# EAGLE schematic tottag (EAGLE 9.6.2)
AUTHOR: Andreas Biri & Pat Pannuto; REV: G; TITLE: TotTag

## Sheet 1 of 4: nRF8240
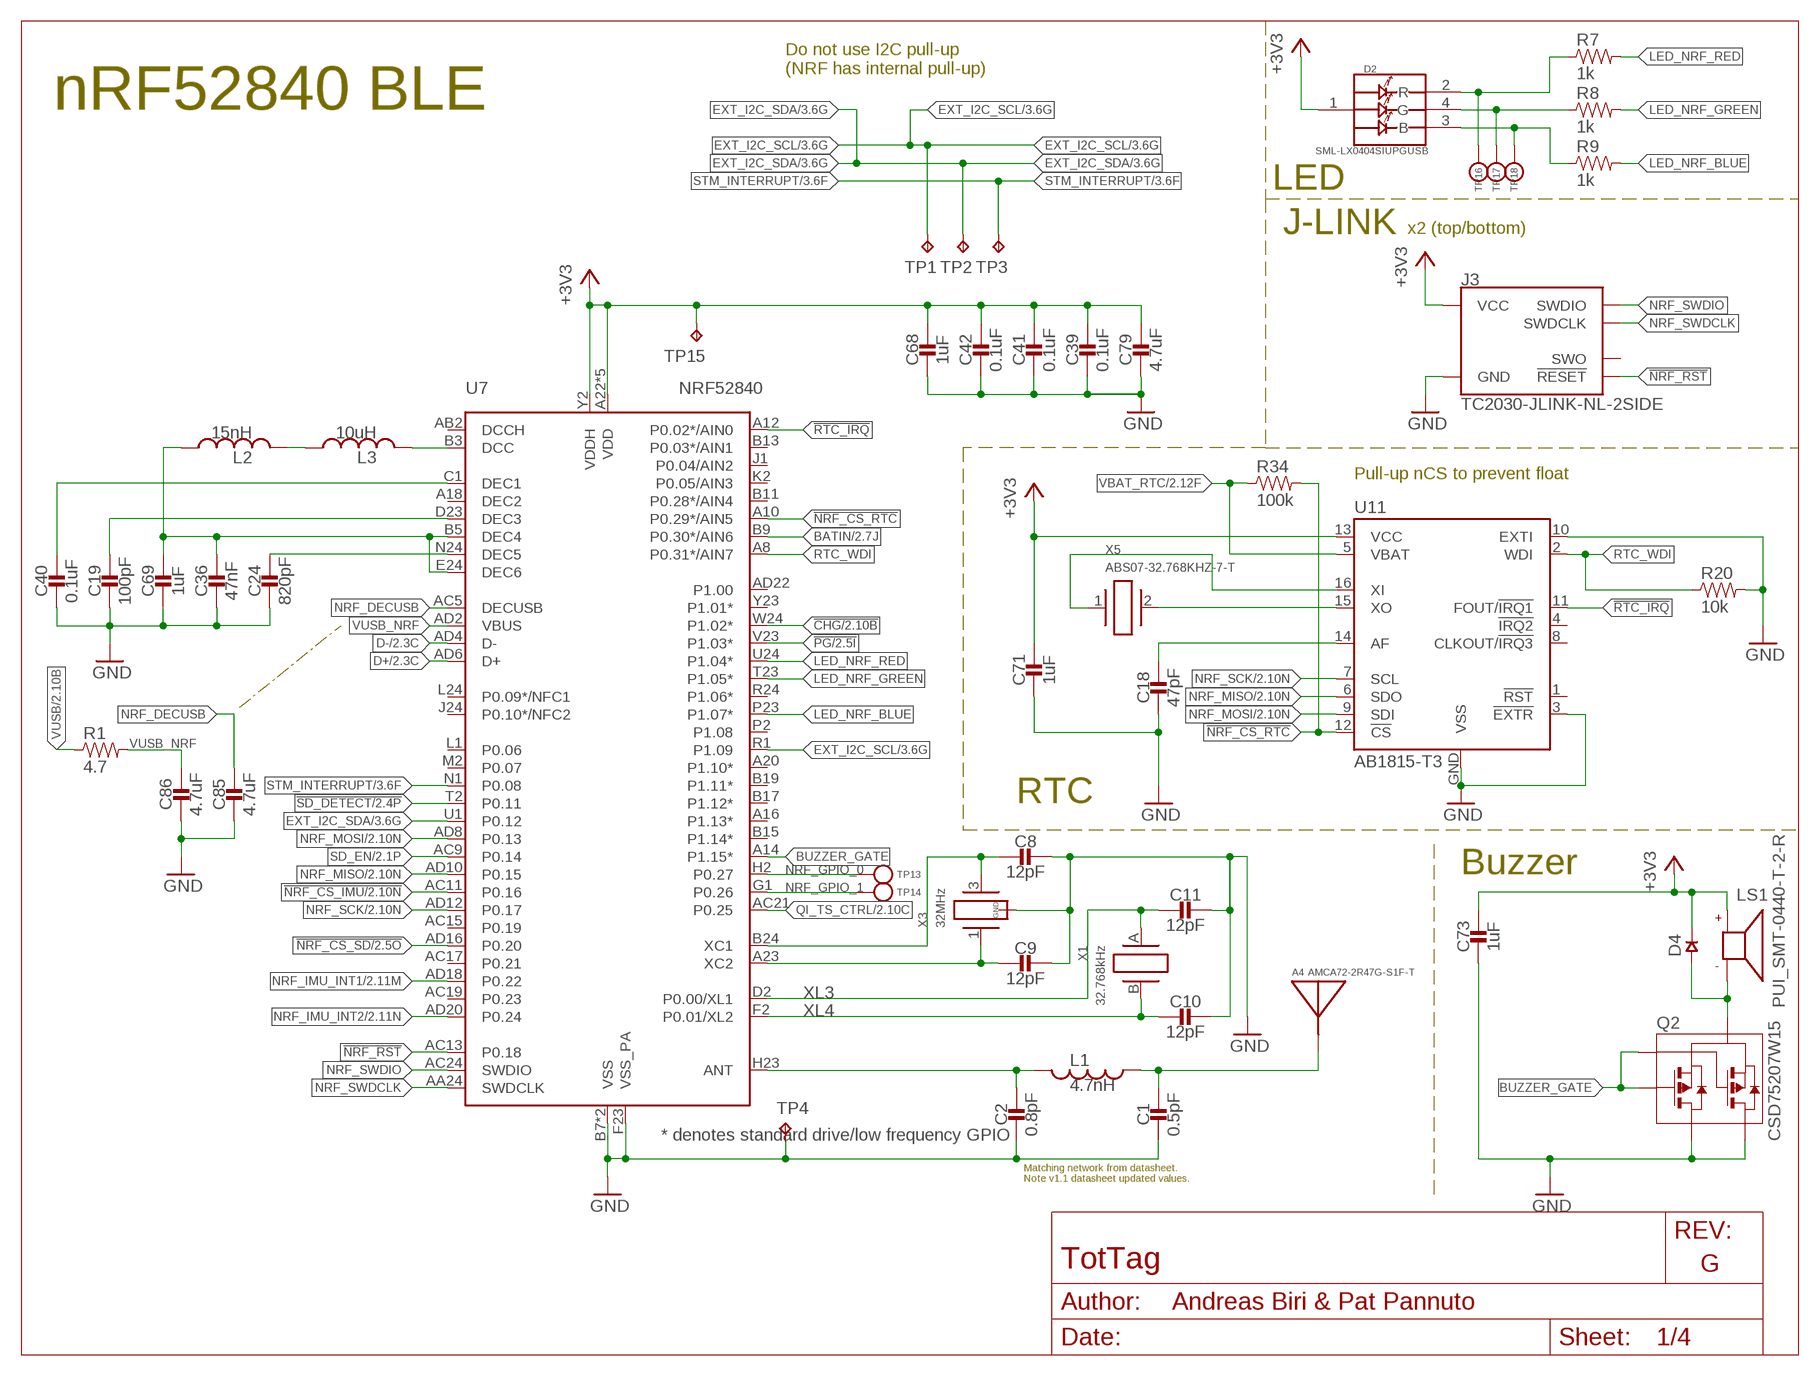
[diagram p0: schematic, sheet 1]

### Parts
A4  AMCA72-2R47G-S1F-T  [AMCA72-2R470G-S1F-T]
C1  0.5pF  CAPACITOR0402_CAP  [0402_CAP]
C2  0.8pF  CAPACITOR0402_CAP  [0402_CAP]
C8  12pF  CAPACITOR0402_CAP  [0402_CAP]
C9  12pF  CAPACITOR0402_CAP  [0402_CAP]
C10  12pF  CAPACITOR0402_CAP  [0402_CAP]
C11  12pF  CAPACITOR0402_CAP  [0402_CAP]
C18  47pF  CAPACITOR0402_CAP  [0402_CAP]
C19  100pF  CAPACITOR0402_CAP  [0402_CAP]
C24  820pF  CAPACITOR0402_CAP  [0402_CAP]
C36  47nF  CAPACITOR0402_CAP  [0402_CAP]
C39  0.1uF  CAPACITOR0402_CAP  [0402_CAP]
C40  0.1uF  CAPACITOR0402_CAP  [0402_CAP]
C41  0.1uF  CAPACITOR0402_CAP  [0402_CAP]
C42  0.1uF  CAPACITOR0402_CAP  [0402_CAP]
C68  1uF  CAPACITOR0402_CAP  [0402_CAP]
C69  1uF  CAPACITOR0402_CAP  [0402_CAP]
C71  1uF  CAPACITOR0402_CAP  [0402_CAP]
C73  1uF  CAPACITOR0402_CAP  [0402_CAP]
C79  4.7uF  CAPACITOR0402_CAP  [0402_CAP]
C85  4.7uF  CAPACITOR0402_CAP  [0402_CAP]
C86  4.7uF  CAPACITOR0402_CAP  [0402_CAP]
D2  SML-LX0404SIUPGUSB  [1MM_SQ_4PAD]
D4  DIODE0402  [0402_DIODE]
J3  TC2030-JLINK-NL-2SIDE  [TC2030-IDC-NL-2SIDE]
L1  4.7nH  INDUCTOR0402  [0402_CAP]
L2  15nH  INDUCTOR0402  [0402_CAP]
L3  10uH  INDUCTOR0603  [0603_CAP]
LS1  PUI_SMT-0440-T-2-R  [SMT-0440-T-2-R]
Q2  CSD75207W15  [DSBGA]
R1  4.7  RESISTOR0402_RES  [0402_RES]
R7  1k  RESISTOR0402_RES  [0402_RES]
R8  1k  RESISTOR0402_RES  [0402_RES]
R9  1k  RESISTOR0402_RES  [0402_RES]
R20  10k  RESISTOR0402_RES  [0402_RES]
R34  100k  RESISTOR0402_RES  [0402_RES]
TP1  TPTP06SQ  [TP06SQ]
TP2  TPTP06SQ  [TP06SQ]
TP3  TPTP06SQ  [TP06SQ]
TP4  TPTP06SQ  [TP06SQ]
TP13  TEST-POINT  [PAD.03X.03]
TP14  TEST-POINT  [PAD.03X.03]
TP15  TPTP06SQ  [TP06SQ]
TP16  TEST-POINT  [PAD.03X.03]
TP17  TEST-POINT  [PAD.03X.03]
TP18  TEST-POINT  [PAD.03X.03]
U7  NRF52840  [AQFN73]
U11  AB1815-T3  [QFN-16-3MM]
X1  32.768kHz  ABS05-32.768KHZ-9-T  [ABS05]
X3  32MHz  7V-32.000MAHV-T  [TXC-7V]
X5  ABS07-32.768KHZ-7-T  [ABS07]

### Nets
!CHG: U7.W24(P1.02*) ; also sheet 2
!NRF_CS_IMU: U7.AC11(P0.16) ; also sheet 2
!NRF_CS_RTC: R34.2 U7.A10(P0.29*/AIN5) U11.12(!CS)
!NRF_CS_SD: U7.AD16(P0.20) ; also sheet 2
!NRF_RST: J3.3(!RESET) J3.B3(!RESET) U7.AC13(P0.18)
!PG: U7.V23(P1.03*) ; also sheet 2
!RTC_IRQ: U7.A12(P0.02*/AIN0) U11.11(FOUT/!IRQ1)
!SD_DETECT: U7.T2(P0.11) ; also sheet 2
+3V3: C39.1 C41.1 C42.1 C68.1 C71.1 C73.1 C79.1 D2.1(VDD) D4.CATHODE J3.1(VCC) J3.B1(VCC) LS1.+(P) TP15.TP U7.A22(VDD) U7.AD14(VDD) U7.AD23(VDD) U7.B1(VDD) U7.W1(VDD) U7.Y2(VDDH) U11.13(VCC) ; also sheet 2,3,4
BATIN: U7.B9(P0.30*/AIN6) ; also sheet 2
BLE_ANT: A4.S1(ANTENNA) C1.1 L1.1
BUZZER_GATE: Q2.A1(G1) Q2.C1(G2) U7.A14(P1.15*)
D+: U7.AD6(D+) ; also sheet 2
D-: U7.AD4(D-) ; also sheet 2
EXT_I2C_SCL: TP1.TP U7.R1(P1.09) ; also sheet 3,4
EXT_I2C_SDA: TP2.TP U7.U1(P0.12) ; also sheet 3,4
GND: C1.2 C2.2 C8.1 C9.1 C10.1 C11.1 C18.2 C19.2 C24.2 C36.2 C39.2 C40.2 C41.2 C42.2 C68.2 C69.2 C71.2 C73.2 C79.2 C85.2 C86.2 J3.5(GND) J3.B5(GND) Q2.A2(D1) Q2.A3(D1) Q2.B2(D2) Q2.B3(D1) Q2.C2(D2) Q2.C3(D2) R20.2 TP4.TP U7.B7(VSS) U7.F23(VSS_PA) U7.GND(VSS) U11.3(!EXTR) U11.10(EXTI) U11.GND(VSS) X3.2(GND) X3.4(GND) ; also sheet 2,3
LED_NRF_BLUE: R9.2 U7.P23(P1.07*)
LED_NRF_GREEN: R8.2 U7.T23(P1.05*)
LED_NRF_RED: R7.2 U7.U24(P1.04*)
N$2: D4.ANODE LS1.-(N) Q2.B1(S)
N$15: C2.1 L1.2 U7.H23(ANT)
N$18: C8.2 U7.B24(XC1) X3.3
N$19: C9.2 U7.A23(XC2) X3.1
N$35: C18.1 U11.14(AF)
N$37: L2.2 L3.1
N$41: U11.16(XI) X5.1
N$42: U11.15(XO) X5.2
N$59: D2.2(R) R7.1 TP16.P$1(TESTPOINT)
N$60: D2.4(G) R8.1 TP17.P$1(TESTPOINT)
N$61: D2.3(B) R9.1 TP18.P$1(TESTPOINT)
NRF_DCC: L3.2 U7.B3(DCC)
NRF_DECAP1: C40.1 U7.C1(DEC1)
NRF_DECAP3: C19.1 U7.D23(DEC3)
NRF_DECAP5: C24.1 U7.N24(DEC5)
NRF_DECAP46: C36.1 C69.1 L2.1 U7.B5(DEC4) U7.E24(DEC6)
NRF_DECUSB: C85.1 U7.AC5(DECUSB)
NRF_GPIO_0: TP13.P$1(TESTPOINT) U7.H2(P0.27)
NRF_GPIO_1: TP14.P$1(TESTPOINT) U7.G1(P0.26)
NRF_IMU_INT1: U7.AD18(P0.22) ; also sheet 2
NRF_IMU_INT2: U7.AD20(P0.24) ; also sheet 2
NRF_MISO: U7.AD10(P0.15) U11.6(SDO) ; also sheet 2
NRF_MOSI: U7.AD8(P0.13) U11.9(SDI) ; also sheet 2
NRF_SCK: U7.AD12(P0.17) U11.7(SCL) ; also sheet 2
NRF_SWDCLK: J3.4(SWDCLK) J3.B4(SWDCLK) U7.AA24(SWDCLK)
NRF_SWDIO: J3.2(SWDIO) J3.B2(SWDIO) U7.AC24(SWDIO)
QI_TS_CTRL: U7.AC21(P0.25) ; also sheet 2
RTC_WDI: R20.1 U7.A8(P0.31*/AIN7) U11.2(WDI)
SD_EN: U7.AC9(P0.14) ; also sheet 2
STM_INTERRUPT: TP3.TP U7.N1(P0.08) ; also sheet 3,4
VBAT_RTC: R34.1 U11.5(VBAT) ; also sheet 2
VUSB: R1.1 ; also sheet 2
VUSB_NRF: C86.1 R1.2 U7.AD2(VBUS)
XL3: C11.2 U7.D2(P0.00/XL1) X1.A
XL4: C10.2 U7.F2(P0.01/XL2) X1.B
Unconnected: J3.6(SWO) J3.B6(SWO) U7.A16(P1.13*) U7.A18(DEC2) U7.A20(P1.10*) U7.AB2(DCCH) U7.AC15(P0.19) U7.AC17(P0.21) U7.AC19(P0.23) U7.AD22(P1.00) U7.B11(P0.28*/AIN4) U7.B13(P0.03*/AIN1) U7.B15(P1.14*) U7.B17(P1.12*) U7.B19(P1.11*) U7.J1(P0.04/AIN2) U7.J24(P0.10*/NFC2) U7.K2(P0.05/AIN3) U7.L1(P0.06) U7.L24(P0.09*/NFC1) U7.M2(P0.07) U7.P2(P1.08) U7.R24(P1.06*) U7.Y23(P1.01*) U11.1(!RST) U11.4(!IRQ2) U11.8(CLKOUT/!IRQ3)

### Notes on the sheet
- Do not use I2C pull-up
  (NRF has internal pull-up)
- nRF52840 BLE
- LED
- J-LINK | x2 (top/bottom)
- Pull-up nCS to prevent float
- RTC
- Buzzer
- Matching network from datasheet.
  Note v1.1 datasheet updated values.

## Sheet 2 of 4: Power + SD + Sensors
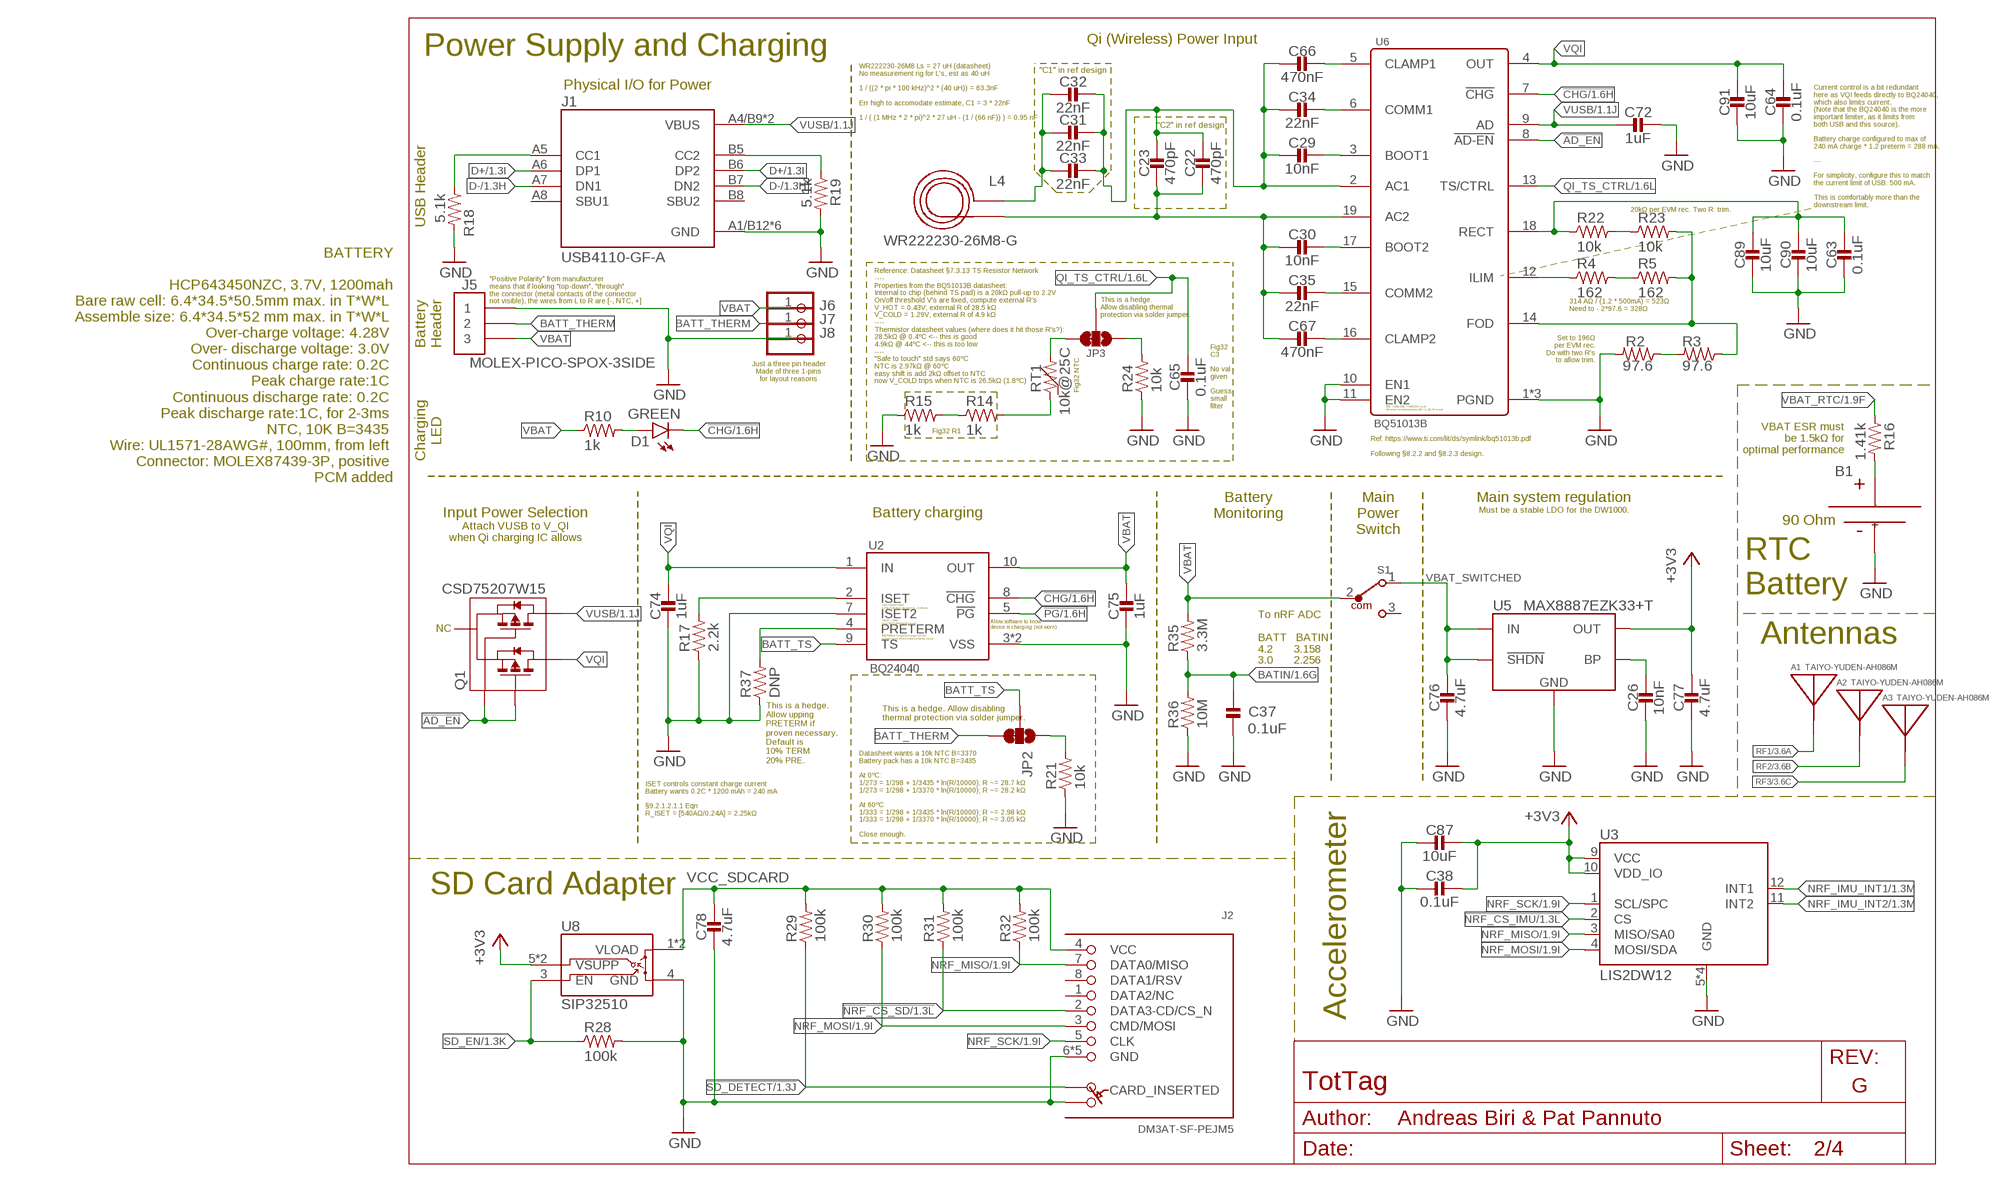
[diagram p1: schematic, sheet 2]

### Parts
A1  TAIYO-YUDEN-AH086M  [TAIYO-YUDEN-AH086M]
A2  TAIYO-YUDEN-AH086M  [TAIYO-YUDEN-AH086M]
A3  TAIYO-YUDEN-AH086M  [TAIYO-YUDEN-AH086M]
B1  MS518SE  [MS518SE-FL35E]
C22  470pF  CAPACITOR0402_CAP  [0402_CAP]
C23  470pF  CAPACITOR0402_CAP  [0402_CAP]
C26  10nF  CAPACITOR0402_CAP  [0402_CAP]
C29  10nF  CAPACITOR0402_CAP  [0402_CAP]
C30  10nF  CAPACITOR0402_CAP  [0402_CAP]
C31  22nF  CAPACITOR0402_CAP  [0402_CAP]
C32  22nF  CAPACITOR0402_CAP  [0402_CAP]
C33  22nF  CAPACITOR0402_CAP  [0402_CAP]
C34  22nF  CAPACITOR0402_CAP  [0402_CAP]
C35  22nF  CAPACITOR0402_CAP  [0402_CAP]
C37  0.1uF  CAPACITOR0402_CAP  [0402_CAP]
C38  0.1uF  CAPACITOR0402_CAP  [0402_CAP]
C63  0.1uF  CAPACITOR0402_CAP  [0402_CAP]
C64  0.1uF  CAPACITOR0402_CAP  [0402_CAP]
C65  0.1uF  CAPACITOR0402_CAP  [0402_CAP]
C66  470nF  CAPACITOR0402_CAP  [0402_CAP]
C67  470nF  CAPACITOR0402_CAP  [0402_CAP]
C72  1uF  CAPACITOR0402_CAP  [0402_CAP]
C74  1uF  CAPACITOR0402_CAP  [0402_CAP]
C75  1uF  CAPACITOR0402_CAP  [0402_CAP]
C76  4.7uF  CAPACITOR0402_CAP  [0402_CAP]
C77  4.7uF  CAPACITOR0402_CAP  [0402_CAP]
C78  4.7uF  CAPACITOR0402_CAP  [0402_CAP]
C87  10uF  CAPACITOR0603_CAP  [0603_CAP]
C89  10uF  CAPACITOR0603_CAP  [0603_CAP]
C90  10uF  CAPACITOR0603_CAP  [0603_CAP]
C91  10uF  CAPACITOR0603_CAP  [0603_CAP]
D1  GREEN  LED0603  [LED-0603]
J1  USB4110-GF-A  [GCT_USB4110-GF-A]
J2  DM3AT-SF-PEJM5  [DM3AT-SF-PEJM5]
J5  MOLEX-PICO-SPOX-3SIDE  [MOLEX-PICO-SPOX-3_SIDE]
J6  PINHD-1X1  [1X01]
J7  PINHD-1X1  [1X01]
J8  PINHD-1X1  [1X01]
JP2  JUMPER-SMT_3_1-NC_TRACE_SILK  [SMT-JUMPER_3_1-NC_TRACE_SILK]
JP3  JUMPER-SMT_3_1-NC_TRACE_SILK  [SMT-JUMPER_3_1-NC_TRACE_SILK]
L4  WR222230-26M8-G  [WR222230-26M8-G]
Q1  CSD75207W15  [DSBGA]
R2  97.6  RESISTOR0402_RES  [0402_RES]
R3  97.6  RESISTOR0402_RES  [0402_RES]
R4  162  RESISTOR0402_RES  [0402_RES]
R5  162  RESISTOR0402_RES  [0402_RES]
R10  1k  RESISTOR0402_RES  [0402_RES]
R14  1k  RESISTOR0402_RES  [0402_RES]
R15  1k  RESISTOR0402_RES  [0402_RES]
R16  1.41k  RESISTOR0402_RES  [0402_RES]
R17  2.2k  RESISTOR0402_RES  [0402_RES]
R18  5.1k  RESISTOR0402_RES  [0402_RES]
R19  5.1k  RESISTOR0402_RES  [0402_RES]
R21  10k  RESISTOR0402_RES  [0402_RES]
R22  10k  RESISTOR0402_RES  [0402_RES]
R23  10k  RESISTOR0402_RES  [0402_RES]
R24  10k  RESISTOR0402_RES  [0402_RES]
R28  100k  RESISTOR0402_RES  [0402_RES]
R29  100k  RESISTOR0402_RES  [0402_RES]
R30  100k  RESISTOR0402_RES  [0402_RES]
R31  100k  RESISTOR0402_RES  [0402_RES]
R32  100k  RESISTOR0402_RES  [0402_RES]
R35  3.3M  RESISTOR0402_RES  [0402_RES]
R36  10M  RESISTOR0402_RES  [0402_RES]
R37  DNP  RESISTOR0402_RES  [0402_RES]
RT1  10k@25C  THERMISTOR0402  [0402_RES]
S1  450404015514  [450404015514]
U2  BQ24040  [DSQ0010A]
U3  LIS2DW12  [LGA-12]
U5  MAX8887EZK33+T  [SOT-23-5]
U6  BQ51013B  [RHL0020A]
U8  SIP32510  [TSOT23-6]

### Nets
!AD_EN: Q1.A1(G1) Q1.C1(G2) U6.8(!AD-EN)
!CHG: D1.C U2.8(!CHG) U6.7(!CHG) ; also sheet 1
!NRF_CS_IMU: U3.2(CS) ; also sheet 1
!NRF_CS_SD: J2.2(DATA3-CD/CS_N) R31.1 ; also sheet 1
!PG: U2.5(!PG) ; also sheet 1
!SD_DETECT: J2.A R29.1 ; also sheet 1
+3V3: C38.1 C77.1 C87.1 U3.9(VCC) U3.10(VDD_IO) U5.5(OUT) U8.5(VSUPP) U8.6(VSUPP) ; also sheet 1,3,4
BATIN: C37.2 R35.1 R36.2 ; also sheet 1
BATT_THERM: J5.2 J5.2SUPP J7.1 JP2.3
BATT_TS: JP2.2 U2.9(TS)
BQ_AC1: C22.1 C23.1 C29.2 C31.1 C32.1 C33.1 C34.2 C66.2 U6.2(AC1)
BQ_AC2: C22.2 C23.2 C30.2 C35.2 C67.2 L4.P$2 U6.19(AC2)
BQ_BOOT1: C29.1 U6.3(BOOT1)
BQ_BOOT2: C30.1 U6.17(BOOT2)
BQ_CLAMP1: C66.1 U6.5(CLAMP1)
BQ_CLAMP2: C67.1 U6.16(CLAMP2)
BQ_COMM1: C34.1 U6.6(COMM1)
BQ_COMM2: C35.1 U6.15(COMM2)
BQ_FOD: R3.1 R5.2 R23.2 U6.14(FOD)
BQ_ILM: R4.1 U6.12(ILIM)
BQ_RECT: C63.1 C89.1 C90.1 R22.1 U6.18(RECT)
COIL_AC1: C31.2 C32.2 C33.2 L4.P$1
D+: J1.A6(DP1) J1.B6(DP2) ; also sheet 1
D-: J1.A7(DN1) J1.B7(DN2) ; also sheet 1
GND: B1.- C26.2 C37.1 C38.2 C63.2 C64.2 C65.2 C72.1 C74.2 C75.2 C76.2 C77.2 C78.2 C87.2 C89.2 C90.2 C91.2 J1.A1/B12(GND) J1.B1/A12(GND) J1.S1(GND) J1.S2(GND) J1.S3(GND) J1.S4(GND) J2.6(GND) J2.B J2.MOUNT0(GND) J2.MOUNT1(GND) J2.MOUNT2(GND) J2.MOUNT3(GND) J5.1 J5.1SUPP J8.1 R2.2 R15.1 R17.1 R18.2 R19.2 R21.1 R24.1 R28.2 R36.1 R37.1 U2.3(VSS) U2.7(ISET2) U2.PAD(VSS) U3.5(GND) U3.6(GND) U3.7(GND) U3.8(GND) U5.2(GND) U6.1(PGND) U6.10(EN1) U6.11(EN2) U6.20(PGND) U6.PAD(PGND) U8.4(GND) ; also sheet 1,3
N$1: J1.B5(CC2) R19.1
N$11: C26.1 U5.4(BP)
N$13: J1.A5(CC1) R18.1
N$28: R2.1 R3.2
N$34: R17.2 U2.2(ISET)
N$45: B1.+ R16.2
N$47: JP2.1 R21.2
N$49: R37.2 U2.4(PRETERM)
N$54: D1.A R10.2
N$64: R22.2 R23.1
N$66: R4.2 R5.1
N$67: JP3.1 R24.2
N$68: JP3.3 RT1.2
N$69: R14.2 RT1.1
N$70: R14.1 R15.2
NRF_IMU_INT1: U3.12(INT1) ; also sheet 1
NRF_IMU_INT2: U3.11(INT2) ; also sheet 1
NRF_MISO: J2.7(DATA0/MISO) R32.1 U3.3(MISO/SA0) ; also sheet 1
NRF_MOSI: J2.3(CMD/MOSI) R30.1 U3.4(MOSI/SDA) ; also sheet 1
NRF_SCK: J2.5(CLK) U3.1(SCL/SPC) ; also sheet 1
QI_TS_CTRL: C65.1 JP3.2 U6.13(TS/CTRL) ; also sheet 1
RF1: A1.A(ANTENNA) ; also sheet 3,4
RF2: A2.A(ANTENNA) ; also sheet 3,4
RF3: A3.A(ANTENNA) ; also sheet 3,4
SD_EN: R28.1 U8.3(EN) ; also sheet 1
VBAT: C75.1 J5.3 J5.3SUPP J6.1 R10.1 R35.2 S1.2 U2.10(OUT)
VBAT_RTC: R16.1 ; also sheet 1
VBAT_SWITCHED: C76.1 S1.1 U5.1(IN) U5.3(!SHDN)
VCC_SDCARD: C78.1 J2.4(VCC) R29.2 R30.2 R31.2 R32.2 U8.1(VLOAD) U8.2(VLOAD)
VQI: C64.1 C74.1 C91.1 Q1.A2(D1) Q1.A3(D1) Q1.B3(D1) U2.1(IN) U6.4(OUT)
VUSB: C72.2 J1.A4/B9(VBUS) J1.B4/A9(VBUS) Q1.B2(D2) Q1.C2(D2) Q1.C3(D2) U6.9(AD) ; also sheet 1
Unconnected: J1.A8(SBU1) J1.B8(SBU2) J2.1(DATA2/NC) J2.8(DATA1/RSV) Q1.B1(S) S1.3

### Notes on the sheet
- Power Supply and Charging | Qi (Wireless) Power Input
- WR222230-26M8 Ls = 27 uH (datasheet)
  No measurement rig for L's, est as 40 uH
  
  1 / ((2 * pi * 100 kHz)^2 * (40 uH)) = 63.3nF
  
  Err high to accomodate estimate, C1 = 3 * 22nF
  
  1 / ( (1 MHz * 2 * pi)^2 * 27 uH - (1 / (66 nF)) ) = 0.95 nF
- "C1" in ref design
- Physical I/O for Power
- "C2" in ref design
- USB Header
- 20kΩ per EVM rec. Two R: trim.
- Current control is a bit redundant
  here as VQI feeds directly to BQ24040,
  which also limits current.
  (Note that the BQ24040 is the more
  important limiter, as it limits from
  both USB and this source).
  
  Battery charge configured to max of
  240 mA charge * 1.2 preterm = 288 mA.
  
  ---
  
  For simplicity, configure this to match
  the current limit of USB: 500 mA.
  
  This is comfortably more than the
  downstream limit.
- BATTERY
  
  HCP643450NZC, 3.7V, 1200mah
  Bare raw cell: 6.4*34.5*50.5mm max. in T*W*L 
  Assemble size: 6.4*34.5*52 mm max. in T*W*L 
  Over-charge voltage: 4.28V 
  Over- discharge voltage: 3.0V 
  Continuous charge rate: 0.2C 
  Peak charge rate:1C 
  Continuous discharge rate: 0.2C 
  Peak discharge rate:1C, for 2-3ms 
  NTC, 10K B=3435 
  Wire: UL1571-28AWG#, 100mm, from left 
  Connector: MOLEX87439-3P, positive 
  PCM added
- Reference: Datasheet §7.3.13 TS Resistor Network
  ----
  Properties from the BQ51013B datasheet:
  Internal to chip (behind TS pad) is a 20kΩ pull-up to 2.2V
  On/off threshold V's are fixed, compute external R's
  V_HOT = 0.43V; external R of 28.5 kΩ
  V_COLD = 1.29V; external R of 4.9 kΩ
  ----
  Thermistor datasheet values (where does it hit those R's?):
  28.5kΩ @ 0.4ºC <-- this is good
  4.9kΩ @ 44ºC <-- this is too low
  ----
  "Safe to touch" std says 60ºC
  NTC is 2.97kΩ @ 60ºC
  easy shift is add 2kΩ offset to NTC
  now V_COLD trips when NTC is 26.5kΩ (1.8ºC)
- This is a hedge.
  Allow disabling thermal
  protection via solder jumper.
- 314 AΩ / (1.2 * 500mA) = 523Ω
  Need to - 2*97.6 = 328Ω
- "Positive Polarity" from manufacturer
  means that if looking "top-down", "through"
  the connector (metal contacts of the connector
  not visible), the wires from L to R are [-, NTC, +]
- Battery
  Header
- Set to 196Ω
  per EVM rec.
  Do with two R's
  to allow trim.
- Fig32
  C3
  
  No val
  given
  
  Guess
  small
  filter
- Just a three pin header
  Made of three 1-pins
  for layout reasons
- Fig32 NTC
- EN1 -> GND, EN2 -> GND [00 case]
  Wireless enabled unless AD > V_AD_Present
- VBAT ESR must
  be 1.5kΩ for
  optimal performance
- Fig32 R1
- Charging
  LED
- Ref: https://www.ti.com/lit/ds/symlink/bq51013b.pdf
  
  Following §8.2.2 and §8.2.3 design.
- Battery
  Monitoring
- Main
  Power
  Switch
- Main system regulation
- Input Power Selection | Battery charging | Must be a stable LDO for the DW1000.
- 90 Ohm
- Attach VUSB to V_QI
  when Qi charging IC allows
- RTC
  Battery
- ISET = KISET / IOUT
  2.25k = 540 AΩ / 240 mA; 2.2k -> 245 mA
- ISET2 -> GND
  Use ISET to limit input current
- Allow software to know
  device is charging (not worn)
- NC
- PRETERM is %age of charge current
  system uses when battery is totally dead
- Antennas
- To nRF ADC
  
  BATT   BATIN
  4.2       3.158
  3.0       2.256
- This is a hedge.
  Allow upping
  PRETERM if
  proven necessary.
  Default is
  10% TERM
  20% PRE.
- This is a hedge. Allow disabling
  thermal protection via solder jumper.
- Datasheet wants a 10k NTC B=3370
  Battery pack has a 10k NTC B=3435
  
  At 0ºC:
  1/273 = 1/298 + 1/3435 * ln(R/10000); R ~= 28.7 kΩ
  1/273 = 1/298 + 1/3370 * ln(R/10000); R ~= 28.2 kΩ
  
  At 60ºC
  1/333 = 1/298 + 1/3435 * ln(R/10000); R ~= 2.98 kΩ
  1/333 = 1/298 + 1/3370 * ln(R/10000); R ~= 3.05 kΩ
  
  Close enough.
- ISET controls constant charge current
  Battery wants 0.2C * 1200 mAh = 240 mA
  
  §9.2.1.2.1.1 Eqn
  R_ISET = [540AΩ/0.24A] = 2.25kΩ
- SD Card Adapter
- Accelerometer

## Sheet 3 of 4: Localization module
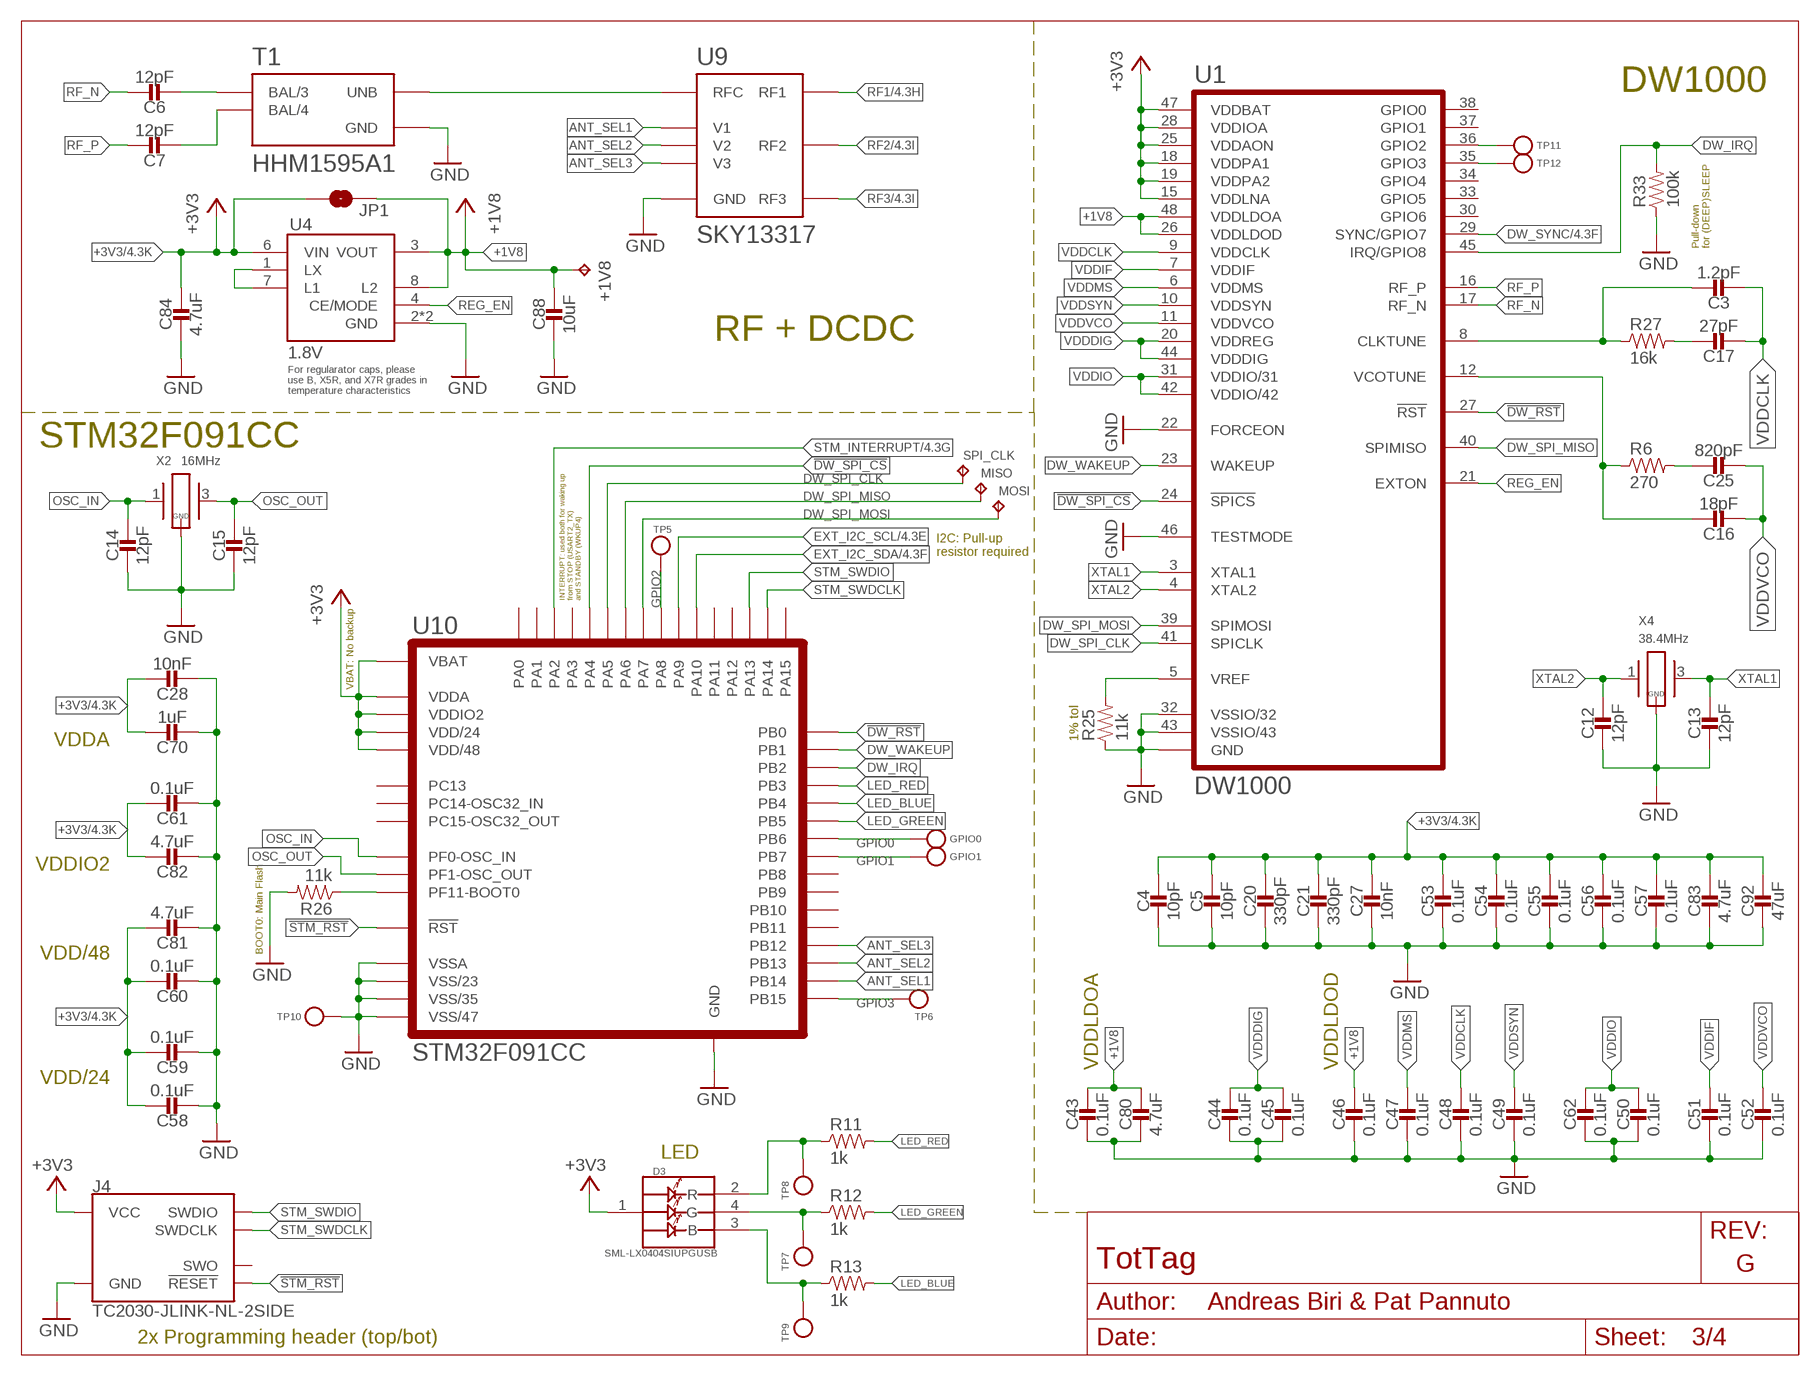
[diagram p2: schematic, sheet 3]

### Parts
+1V8  TPTP06SQ  [TP06SQ]
C3  1.2pF  CAPACITOR0402_CAP  [0402_CAP]
C4  10pF  CAPACITOR0402_CAP  [0402_CAP]
C5  10pF  CAPACITOR0402_CAP  [0402_CAP]
C6  12pF  CAPACITOR0201_CAP  [0201_CAP]
C7  12pF  CAPACITOR0201_CAP  [0201_CAP]
C12  12pF  CAPACITOR0402_CAP  [0402_CAP]
C13  12pF  CAPACITOR0402_CAP  [0402_CAP]
C14  12pF  CAPACITOR0402_CAP  [0402_CAP]
C15  12pF  CAPACITOR0402_CAP  [0402_CAP]
C16  18pF  CAPACITOR0402_CAP  [0402_CAP]
C17  27pF  CAPACITOR0402_CAP  [0402_CAP]
C20  330pF  CAPACITOR0402_CAP  [0402_CAP]
C21  330pF  CAPACITOR0402_CAP  [0402_CAP]
C25  820pF  CAPACITOR0402_CAP  [0402_CAP]
C27  10nF  CAPACITOR0402_CAP  [0402_CAP]
C28  10nF  CAPACITOR0402_CAP  [0402_CAP]
C43  0.1uF  CAPACITOR0402_CAP  [0402_CAP]
C44  0.1uF  CAPACITOR0402_CAP  [0402_CAP]
C45  0.1uF  CAPACITOR0402_CAP  [0402_CAP]
C46  0.1uF  CAPACITOR0402_CAP  [0402_CAP]
C47  0.1uF  CAPACITOR0402_CAP  [0402_CAP]
C48  0.1uF  CAPACITOR0402_CAP  [0402_CAP]
C49  0.1uF  CAPACITOR0402_CAP  [0402_CAP]
C50  0.1uF  CAPACITOR0402_CAP  [0402_CAP]
C51  0.1uF  CAPACITOR0402_CAP  [0402_CAP]
C52  0.1uF  CAPACITOR0402_CAP  [0402_CAP]
C53  0.1uF  CAPACITOR0402_CAP  [0402_CAP]
C54  0.1uF  CAPACITOR0402_CAP  [0402_CAP]
C55  0.1uF  CAPACITOR0402_CAP  [0402_CAP]
C56  0.1uF  CAPACITOR0402_CAP  [0402_CAP]
C57  0.1uF  CAPACITOR0402_CAP  [0402_CAP]
C58  0.1uF  CAPACITOR0402_CAP  [0402_CAP]
C59  0.1uF  CAPACITOR0402_CAP  [0402_CAP]
C60  0.1uF  CAPACITOR0402_CAP  [0402_CAP]
C61  0.1uF  CAPACITOR0402_CAP  [0402_CAP]
C62  0.1uF  CAPACITOR0402_CAP  [0402_CAP]
C70  1uF  CAPACITOR0402_CAP  [0402_CAP]
C80  4.7uF  CAPACITOR0402_CAP  [0402_CAP]
C81  4.7uF  CAPACITOR0402_CAP  [0402_CAP]
C82  4.7uF  CAPACITOR0402_CAP  [0402_CAP]
C83  4.7uF  CAPACITOR0402_CAP  [0402_CAP]
C84  4.7uF  CAPACITOR0402_CAP  [0402_CAP]
C88  10uF  CAPACITOR0603_CAP  [0603_CAP]
C92  47uF  CAPACITOR0603_CAP  [0603_CAP]
D3  SML-LX0404SIUPGUSB  [1MM_SQ_4PAD]
GPIO0  TEST-POINT  [PAD.03X.03]
GPIO1  TEST-POINT  [PAD.03X.03]
J4  TC2030-JLINK-NL-2SIDE  [TC2030-IDC-NL-2SIDE]
JP1  JUMPER-SMT_2_NO_SILK  [SMT-JUMPER_2_NO_SILK]
MISO  TPTP06SQ  [TP06SQ]
MOSI  TPTP06SQ  [TP06SQ]
R6  270  RESISTOR0402_RES  [0402_RES]
R11  1k  RESISTOR0402_RES  [0402_RES]
R12  1k  RESISTOR0402_RES  [0402_RES]
R13  1k  RESISTOR0402_RES  [0402_RES]
R25  11k  RESISTOR0402_RES  [0402_RES]
R26  11k  RESISTOR0402_RES  [0402_RES]
R27  16k  RESISTOR0402_RES  [0402_RES]
R33  100k  RESISTOR0402_RES  [0402_RES]
SPI_CLK  TPTP06SQ  [TP06SQ]
T1  HHM1595A1  [EIA-0805]
TP5  TEST-POINT  [PAD.03X.03]
TP6  TEST-POINT  [PAD.03X.03]
TP7  TEST-POINT  [PAD.03X.03]
TP8  TEST-POINT  [PAD.03X.03]
TP9  TEST-POINT  [PAD.03X.03]
TP10  TEST-POINT  [PAD.03X.03]
TP11  TEST-POINT  [PAD.03X.03]
TP12  TEST-POINT  [PAD.03X.03]
U1  DW1000  [QFN-48-DW1000]
U4  1.8V  XCL206B  [XCL20X]
U9  SKY13317  [MLPQ-UT-8]
U10  STM32F091CC  [UFQFPN-48]
X2  16MHz  FA-20H  [FA-20H]
X4  38.4MHz  FA-20H  [FA-20H]

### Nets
!DW_RST: U1.27(!RST) U10.18(PB0)
!DW_SPI_CS: U1.24(!SPICS) U10.14(PA4)
!STM_RST: J4.3(!RESET) J4.B3(!RESET) U10.7(!RST)
+1V8: +1V8.TP C43.1 C46.1 C80.1 C88.1 JP1.2 U1.26(VDDLDOD) U1.48(VDDLDOA) U4.3(VOUT) U4.8(L2)
+3V3: C4.1 C5.1 C20.1 C21.1 C27.1 C28.1 C53.1 C54.1 C55.1 C56.1 C57.1 C58.1 C59.1 C60.1 C61.1 C70.1 C81.1 C82.1 C83.1 C84.1 C92.1 D3.1(VDD) J4.1(VCC) J4.B1(VCC) JP1.1 U1.15(VDDLNA) U1.18(VDDPA1) U1.19(VDDPA2) U1.25(VDDAON) U1.28(VDDIOA) U1.47(VDDBAT) U4.6(VIN) U10.1(VBAT) U10.9(VDDA) U10.24(VDD/24) U10.36(VDDIO2) U10.48(VDD/48) ; also sheet 1,2,4
ANT_SEL1: U9.3(V1) U10.27(PB14)
ANT_SEL2: U9.6(V2) U10.26(PB13)
ANT_SEL3: U9.7(V3) U10.25(PB12)
DW_IRQ: R33.2 U1.45(IRQ/GPIO8) U10.20(PB2)
DW_SPI_CLK: SPI_CLK.TP U1.41(SPICLK) U10.15(PA5)
DW_SPI_MISO: MISO.TP U1.40(SPIMISO) U10.16(PA6)
DW_SPI_MOSI: MOSI.TP U1.39(SPIMOSI) U10.17(PA7)
DW_SYNC: U1.29(SYNC/GPIO7) ; also sheet 4
DW_WAKEUP: U1.23(WAKEUP) U10.19(PB1)
EXT_I2C_SCL: U10.30(PA9) ; also sheet 1,4
EXT_I2C_SDA: U10.31(PA10) ; also sheet 1,4
GND: C4.2 C5.2 C12.2 C13.2 C14.2 C15.2 C20.2 C21.2 C27.2 C28.2 C43.2 C44.2 C45.2 C46.2 C47.2 C48.2 C49.2 C50.2 C51.2 C52.2 C53.2 C54.2 C55.2 C56.2 C57.2 C58.2 C59.2 C60.2 C61.2 C62.2 C70.2 C80.2 C81.2 C82.2 C83.2 C84.2 C88.2 C92.2 J4.5(GND) J4.B5(GND) R25.1 R26.2 R33.1 T1.2(GND) T1.5(GND) TP10.P$1(TESTPOINT) U1.22(FORCEON) U1.32(VSSIO/32) U1.43(VSSIO/43) U1.46(TESTMODE) U1.GND U4.2(GND) U4.5(GND) U9.GND U10.8(VSSA) U10.23(VSS/23) U10.35(VSS/35) U10.47(VSS/47) U10.GND X2.2(GND) X2.4(GND) X4.2(GND) X4.4(GND) ; also sheet 1,2
GPIO0: GPIO0.P$1(TESTPOINT) U10.42(PB6)
GPIO1: GPIO1.P$1(TESTPOINT) U10.43(PB7)
GPIO2: TP5.P$1(TESTPOINT) U10.29(PA8)
GPIO3: TP6.P$1(TESTPOINT) U10.28(PB15)
LED_BLUE: R13.2 U10.40(PB4)
LED_GREEN: R12.2 U10.41(PB5)
LED_RED: R11.2 U10.39(PB3)
N$3: T1.1(UNB) U9.1(RFC)
N$4: C6.P$2 T1.3(BAL/3)
N$7: C7.P$2 T1.4(BAL/4)
N$8: C25.1 R6.2
N$12: C17.1 R27.2
N$14: C16.1 R6.1 U1.12(VCOTUNE)
N$16: C3.1 R27.1 U1.8(CLKTUNE)
N$21: R25.2 U1.5(VREF)
N$22: R26.1 U10.44(PF11-BOOT0)
N$23: D3.4(G) R12.1 TP7.P$1(TESTPOINT)
N$24: D3.3(B) R13.1 TP9.P$1(TESTPOINT)
N$25: D3.2(R) R11.1 TP8.P$1(TESTPOINT)
N$26: TP11.P$1(TESTPOINT) U1.36(GPIO2)
N$27: TP12.P$1(TESTPOINT) U1.35(GPIO3)
N$44: U4.1(LX) U4.7(L1)
OSC_IN: C14.1 U10.5(PF0-OSC_IN) X2.1
OSC_OUT: C15.1 U10.6(PF1-OSC_OUT) X2.3
REG_EN: U1.21(EXTON) U4.4(CE/MODE)
RF1: U9.4(RF1) ; also sheet 2,4
RF2: U9.5(RF2) ; also sheet 2,4
RF3: U9.8(RF3) ; also sheet 2,4
RF_N: C6.P$1 U1.17(RF_N)
RF_P: C7.P$1 U1.16(RF_P)
STM_INTERRUPT: U10.12(PA2) ; also sheet 1,4
STM_SWDCLK: J4.4(SWDCLK) J4.B4(SWDCLK) U10.37(PA14)
STM_SWDIO: J4.2(SWDIO) J4.B2(SWDIO) U10.34(PA13)
VDDCLK: C3.2 C17.2 C48.1 U1.9(VDDCLK)
VDDDIG: C44.1 C45.1 U1.20(VDDREG) U1.44(VDDDIG)
VDDIF: C51.1 U1.7(VDDIF)
VDDIO: C50.1 C62.1 U1.31(VDDIO/31) U1.42(VDDIO/42)
VDDMS: C47.1 U1.6(VDDMS)
VDDSYN: C49.1 U1.10(VDDSYN)
VDDVCO: C16.2 C25.2 C52.1 U1.11(VDDVCO)
XTAL1: C13.1 U1.3(XTAL1) X4.3
XTAL2: C12.1 U1.4(XTAL2) X4.1
Unconnected: J4.6(SWO) J4.B6(SWO) U1.30(GPIO6) U1.33(GPIO5) U1.34(GPIO4) U1.37(GPIO1) U1.38(GPIO0) U10.2(PC13) U10.3(PC14-OSC32_IN) U10.4(PC15-OSC32_OUT) U10.10(PA0) U10.11(PA1) U10.13(PA3) U10.21(PB10) U10.22(PB11) U10.32(PA11) U10.33(PA12) U10.38(PA15) U10.45(PB8) U10.46(PB9)

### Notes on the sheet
- DW1000
- Pull-down
  for (DEEP)SLEEP
- RF + DCDC
- For regularator caps, please
  use B, X5R, and X7R grades in
  temperature characteristics
- STM32F091CC
- I2C: Pull-up
  resistor required
- INTERRUPT: used both for waking up
  from STOP (USART2_TX)
  and STANDBY (WKUP4)
- VBAT: No backup
- VDDA
- 1% tol
- VDDIO2
- VDD/48
- BOOT0: Main Flash
- VDD/24 | VDDLDOA | VDDLDOD
- LED
- 2x Programming header (top/bot)

## Sheet 4 of 4: External signals
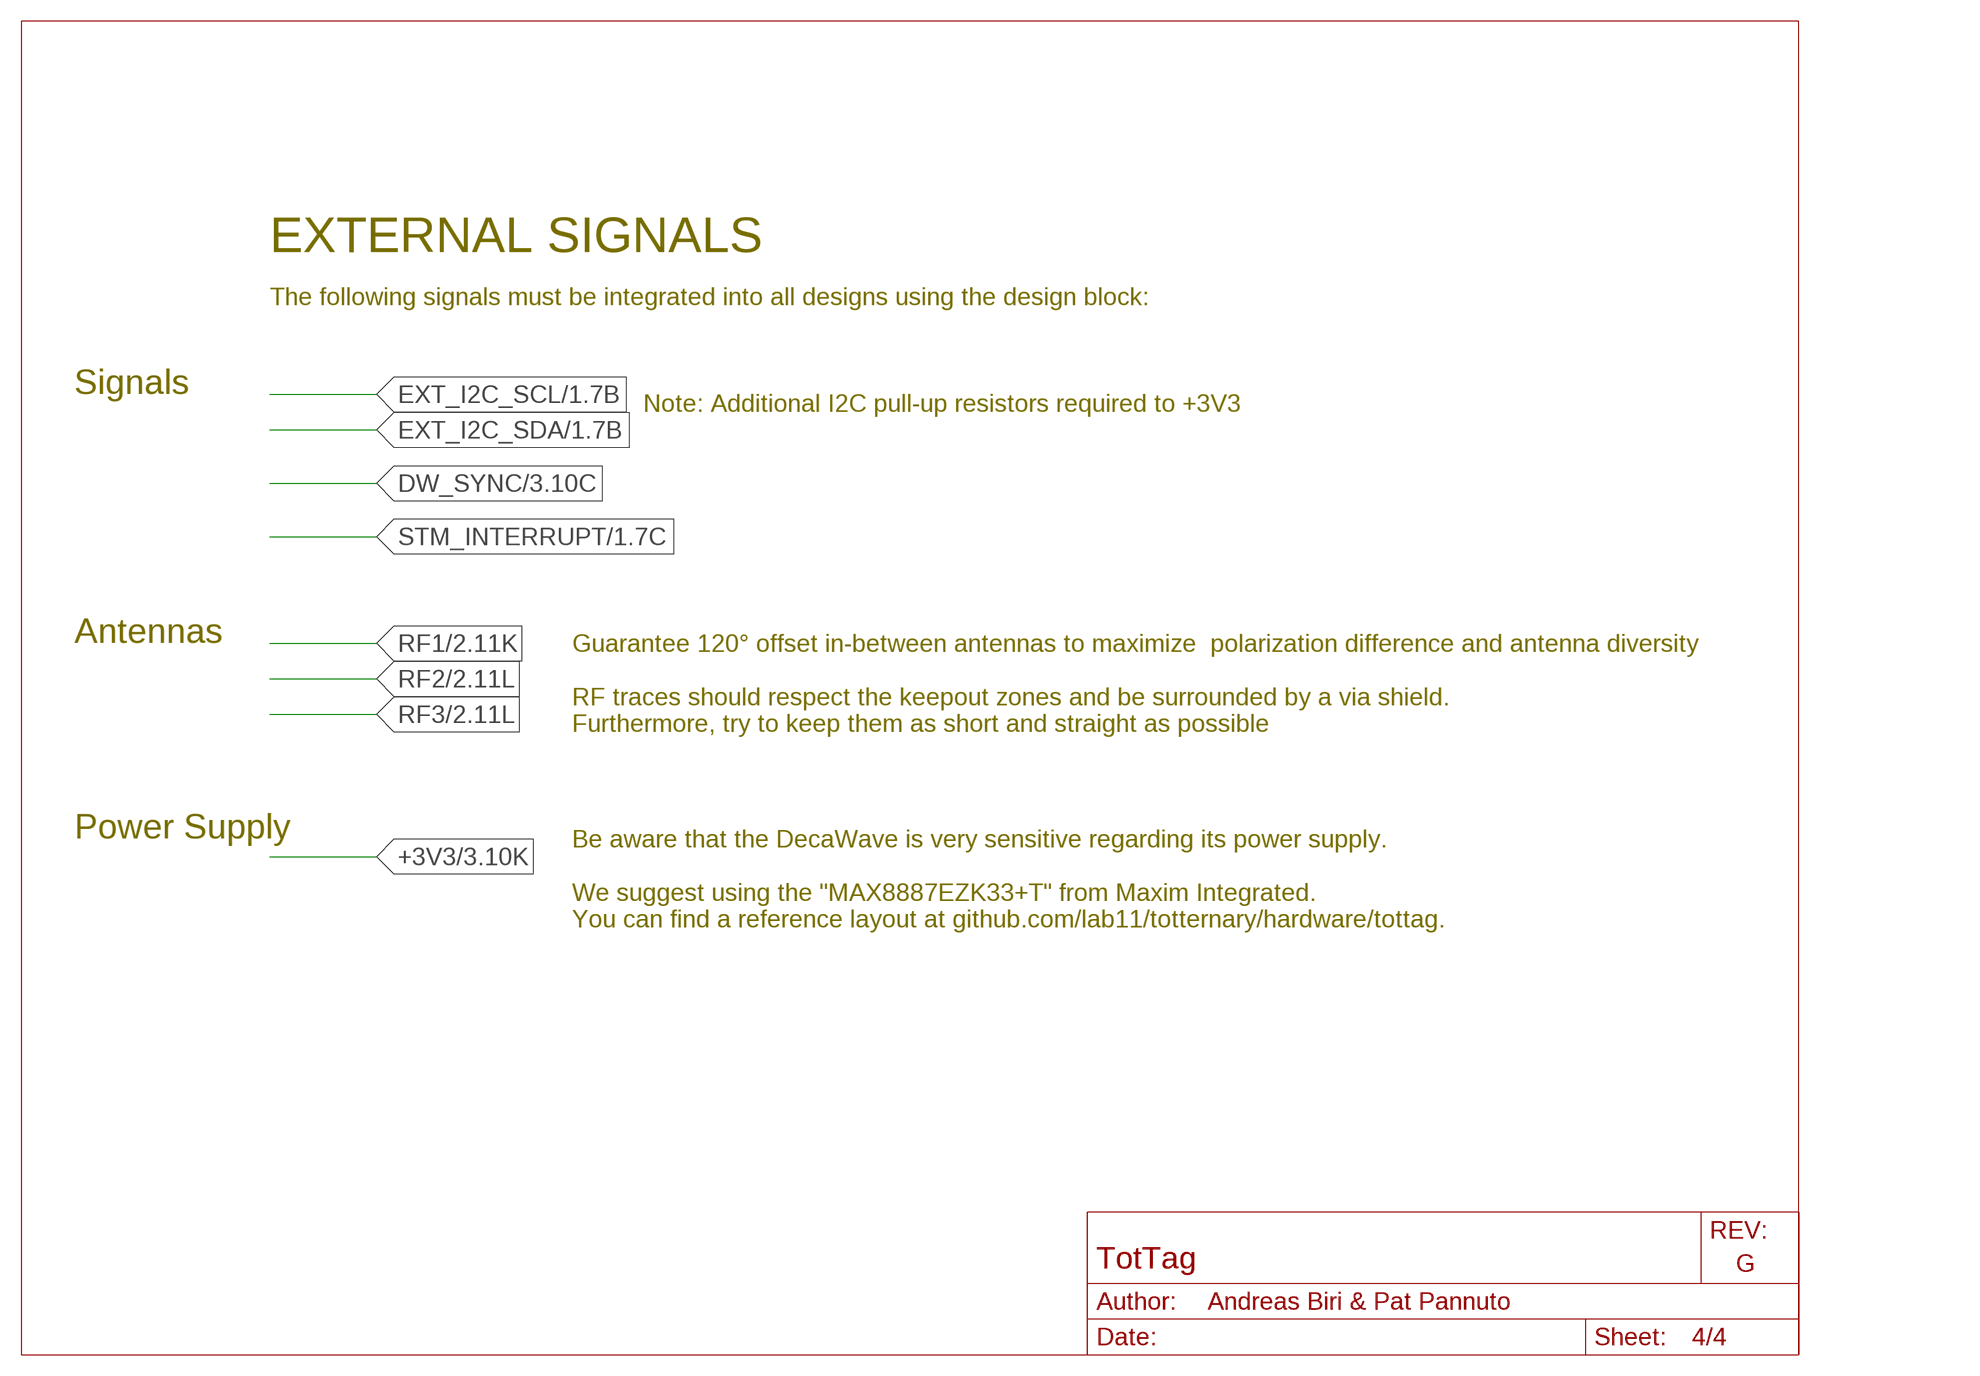
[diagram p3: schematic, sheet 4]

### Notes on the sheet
- EXTERNAL SIGNALS
- The following signals must be integrated into all designs using the design block:
- Signals
- Note: Additional I2C pull-up resistors required to +3V3
- Antennas
- Guarantee 120° offset in-between antennas to maximize  polarization difference and antenna diversity
  
  RF traces should respect the keepout zones and be surrounded by a via shield. 
  Furthermore, try to keep them as short and straight as possible
- Power Supply
- Be aware that the DecaWave is very sensitive regarding its power supply.
  
  We suggest using the "MAX8887EZK33+T" from Maxim Integrated.
  You can find a reference layout at github.com/lab11/totternary/hardware/tottag.

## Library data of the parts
+1V8 MISO MOSI SPI_CLK TP1-TP4 TP15 = testpad:TP: Test pad
A1-A3 = antennas:TAIYO-YUDEN-AH086M: UWB Antenna - 3.1-8GHz; DIGIKEY: 587-2204-1-ND; MPN: AH086M555003-T
A4 = antennas:AMCA72-2R47G-S1F-T: WiFi/Bluetooth/ZigBee, ISM Atenna; DESCRIPTION: RF ANT 2.4GHZ CHIP SOLDER SMD; DIGIKEY: 535-14108-1-ND; MPN: AMCA72-2R470G-S1F-T4
B1 = batteries:MS518SE: A small, low leakage rechargeable battery for RTC backup; DIGIKEY: 728-1054-ND; MANUFACTURER: Seiko; MPN: MS518SE-FL35E
C1 = passives:CAPACITOR: SMD Capacitor; DIGIKEY: 490-11250-1-ND; MPN: GJM1555C1HR50WB01D
C2 = passives:CAPACITOR: SMD Capacitor; DIGIKEY: 490-11253-1-ND; MPN: GJM1555C1HR80WB01D
C3 = passives:CAPACITOR: SMD Capacitor; DIGIKEY: 490-3085-1-ND; MPN: GJM1555C1H1R2CB01D
C4 C5 = passives:CAPACITOR: SMD Capacitor; DIGIKEY: 732-12054-1-ND; MPN: 885012005074
C6 C7 = passives:CAPACITOR: SMD Capacitor; DIGIKEY: 399-8604-2-ND; MPN: CBR02C120F3GAC
C8-C15 = passives:CAPACITOR: SMD Capacitor; DIGIKEY: 399-8815-2-ND; MPN: CBR04C120F5GAC
C16 = passives:CAPACITOR: SMD Capacitor; DIGIKEY: 399-8828-1-ND; MPN: CBR04C180F5GAC
C17 = passives:CAPACITOR: SMD Capacitor; DIGIKEY: 490-16380-1-ND; MPN: GJM1555C1H270FB01D
C18 = passives:CAPACITOR: SMD Capacitor; DIGIKEY: 490-5942-1-ND; MPN: GRM1555C1H470JA01D
C19 = passives:CAPACITOR: SMD Capacitor; DIGIKEY: 490-5922-1-ND; MPN: GRM1555C1H101JA01D
C20 C21 = passives:CAPACITOR: SMD Capacitor; DIGIKEY: 311-3768-1-ND; MPN: CC0402JRX7R9BB331
C22 C23 = passives:CAPACITOR: SMD Capacitor; DESCRIPTION: CAP CER 470PF 50V C0G/NP0 0402; DIGIKEY: 490-6242-1-ND; MANUFACTURER: Murata; MPN: GRM1555C1H471JA01J
C24 C25 = passives:CAPACITOR: SMD Capacitor; DIGIKEY: 399-11129-2-ND; MPN: C0402C821J5GACTU
C26-C28 C37 C42-C62 C68 C70 C72 C76 C77 C79-C84 = passives:CAPACITOR: SMD Capacitor
C29 C30 = passives:CAPACITOR: SMD Capacitor; DIGIKEY: 490-6351-2-ND; MPN: GRM155R71H103KA88J
C31-C33 = passives:CAPACITOR: SMD Capacitor; DIGIKEY: 490-10699-2-ND; MPN: GRM155R71E223JA61D
C34 C35 = passives:CAPACITOR: SMD Capacitor; DIGIKEY: 311-3823-1-ND; MPN: CC0402ZRY5V8BB223
C36 = passives:CAPACITOR: SMD Capacitor; DIGIKEY: 445-1264-1-ND; MPN: C1005X7R1C473K050BC
C38-C41 C63-C65 = passives:CAPACITOR: SMD Capacitor; DIGIKEY: 490-6328-1-ND; MPN: GRM155R71C104KA88J
C66 C67 = passives:CAPACITOR: SMD Capacitor; DIGIKEY: 490-12270-1-ND; MPN: GRT155R61E474ME01D
C69 C71 C73-C75 = passives:CAPACITOR: SMD Capacitor; DIGIKEY: 490-7195-1-ND; MPN: GRM155R70G105KA12D
C78 C85 C86 = passives:CAPACITOR: SMD Capacitor; DESCRIPTION: CAP CER 4.7UF 6.3V X5R 0402; DIGIKEY: 445-5947-1-ND; MANUFACTURER: TDK; MPN: C1005X5R0J475K050BC
C87-C91 = passives:CAPACITOR: SMD Capacitor; DIGIKEY: 1253-CM105X5R106M25ATCT-ND; MPN: CM105X5R106M25AT
C92 = passives:CAPACITOR: SMD Capacitor; DIGIKEY: 490-13247-1-ND; MPN: GRM188R60J476ME15D
D1 = SparkFun-LED:LED: LED (Generic); DIGIKEY: 160-1446-1-ND; MPN: LTST-C191KGKT
D2 D3 = leds:SML-LX0404SIUPGUSB: 1mm^2 RGB LED; DIGIKEY: 67-2125-1-ND; MANUFACTURER: Lumex Opto; MPN: SML-LX0404SIUPGUSB
D4 = passives:DIODE; DIGIKEY: 641-2087-1-ND; MPN: CDSQR400B-HF
GPIO0 GPIO1 TP5-TP14 TP16-TP18 = headers:TEST-POINT
J1 = connector:USB4110-GF-A: CONN USB 2.0 TYPE-C R/A SMT; DESCRIPTION: USB-C (USB TYPE-C) USB 2.0 Receptacle Connector 24 (16+8 Dummy) Position Surface Mount, Right Angle; Through Hole; DIGIKEY: 2073-USB4110-GF-A-1-ND; MF: GCT; MPN: USB4110-GF-A; PACKAGE: None
J2 = connector:DM3AT-SF-PEJM5: CONN MICRO SD R/A PUSH-PUSH SMD; DESCRIPTION: CONN MICRO SD CARD PUSH-PUSH R/A; DIGIKEY: HR1964CT-ND; MANUFACTURER: Hirose Electric Co Ltd; MPN: DM3AT-SF-PEJM5
J3 J4 = connector:TC2030-JLINK
J5 = connector:MOLEX-PICO-SPOX-3: MOLEX 1.50mm Pitch, Pico-SPOX PCB Header, Single Row, Surface Mount. Default connector of Shenzhen LiPo + Thermistor suppliers ca. 2020.; DIGIKEY: WM7647CT-ND; MFN: 874380343
J6-J8 = pinhead:PINHD-1X1: PIN HEADER
JP1 = SparkFun-Jumpers:JUMPER-SMT_2_NO: Normally open jumper
JP2 JP3 = SparkFun-Jumpers:JUMPER-SMT_3_1-NC_TRACE: Normally closed trace jumper (1 of 2 connections) This jumper has a trace between two pads so it's normally closed (NC). The other connection is normally open (NO). Use a razor knife to open the connection. For best results follow the IPC guidelines for cutting traces: Cutout at least 0.063 mm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
L1 = passives:INDUCTOR: A very specific inductor; DIGIKEY: 490-15482-1-ND; MPN: LQW15AN4N7G8ZD
L2 = passives:INDUCTOR: A very specific inductor; DIGIKEY: 587-1521-1-ND; MPN: HK100515NJ-T
L3 = passives:INDUCTOR: A very specific inductor; DIGIKEY: 490-4025-1-ND; MPN: LQM18FN100M00D
L4 = ac:WR222230-26M8-G: Small Rx Coil for Wireless Power Transfer.; DIGIKEY: 445-173093-ND; MPN: WR222230-26M8-G
LS1 = audio:PUI_SMT-0440-T-2-R; DIGIKEY: 668-SMT-0440-T-2-RTR-ND; MPN: SMT-0440-T-2-R
Q1 Q2 = fets:CSD75207W15: low on resistance, gate charge dual p-channel nexfet; DIGIKEY: 296-40008-1-ND; MANUFACTURER: TEXAS INSTRUMENTS; MPN: CSD75207W15
R1 = passives:RESISTOR: Resistor; DIGIKEY: RMCF0402FT4R70CT-ND; MPN: RMCF0402FT4R70
R2 R3 = passives:RESISTOR: Resistor; DIGIKEY: RMCF0402FT97R6CT-ND; MPN: RMCF0402FT97R6
R4 R5 = passives:RESISTOR: Resistor; DIGIKEY: RMCF0402FT162RCT-ND; MPN: RMCF0402FT162R
R6 = passives:RESISTOR: Resistor; DIGIKEY: RMCF0402FT270RCT-ND; MPN: RMCF0402FT270R
R7 = passives:RESISTOR: Resistor; DIGIKEY: RMCF0402FT1K00CT-ND; MPN: RMCF0402FT1K00
R8-R15 R28-R34 R37 = passives:RESISTOR: Resistor
R16 = passives:RESISTOR: Resistor; DIGIKEY: RMCF0402FT1K40CT-ND; MPN: RMCF0402FT1K40
R17 = passives:RESISTOR: Resistor; DIGIKEY: RMCF0402JT2K20CT-ND; MPN: RMCF0402JT2K20
R18 R19 = passives:RESISTOR: Resistor; DIGIKEY: RMCF0402FT5K10CT-ND; MPN: RMCF0402FT5K10
R20-R24 = passives:RESISTOR: Resistor; DIGIKEY: 311-10KJRCT-ND; MPN: RC0402JR-0710KL
R25 R26 = passives:RESISTOR: Resistor; DIGIKEY: RMCF0402FT11K0CT-ND; MPN: RMCF0402FT11K0
R27 = passives:RESISTOR: Resistor; DIGIKEY: RMCF0402FT16K0CT-ND; MPN: RMCF0402FT16K0
R35 = passives:RESISTOR: Resistor; DIGIKEY: RMCF0402FT3M30CT-ND; MPN: RMCF0402FT3M30
R36 = passives:RESISTOR: Resistor; DIGIKEY: RMCF0402FT10M0CT-ND; MPN: RMCF0402FT10M0
RT1 = passives:THERMISTOR: Thermistor.; DIGIKEY: 490-18149-1-ND; MPN: NCU15XH103F60RC
S1 = Wurth_Switch_WS-SLSU:450404015514: WS-SLSU Mini Slide Switch, Same Side Connection Side Push 6.7x2.7 mm Properties Actuator Material:PA46 Actuator Flammability Rating:UL94 HB Actuator Color:Black Frame Material:LCP Frame Flammability Rating:UL94 V-0 Frame Color:Black Contact Material:Copper Alloy Contact Plating:Silver Terminal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; DATASHEET-URL: https://www.we-online.com/catalog/datasheet/450404015514.pdf; DIGIKEY: 732-13665-1-ND; IR: 300mA; PACKAGING: Tape and Reel; PART-NUMBER: 450404015514; QTY: 150; VR: 5V(DC)
T1 = rf:HHM1595A1: Description: Symbol for HHM1595A1, a multilayer Balun from TDK.; DATASHEET: https://product.tdk.com/info/en/documents/data_sheet/rf_balun_hhm1595a1_en.pdf; DESCRIPTION: XFMR BALUN RF 3.0-8.0GHZ UWB SMD; DIGIKEY: 445-3387-1-ND; MANUFACTURER: TDK Corporation; MOUSER: 810-HHM1595A1; MPN: HHM1595A1
U1 = chips:DW1000: Description: The DecaWave DW1000 chip, used for UWB two-way ranging.; DATASHEET: https://www.decawave.com/sites/default/files/resources/dw1000-datasheet-v2.13.pdf; DESCRIPTION: IC RF TXRX 802.15.4 48-QFN; DIGIKEY: 1479-1001-1-ND; MANUFACTURER: Decawave Limited; MPN: DW1000-I-TR13
U2 = chips:BQ24040: Simple Li Ion / Li Poly charger.; DIGIKEY: 296-37142-1-ND; MPN: BQ24040
U3 = chips:LIS2DW12: ultra low power 3 axis accelerometer; DIGIKEY: 497-17718-6-ND; MANUFACTURER: STMicroelectronics; MOUSER: 511-LIS2DW12TR; MPN: LIS2DW12TR
U4 = regulators:XCL206: Non-Isolated PoL Module DC DC Converter 1 Output 1.8V 600mA 2V - 6V Input; DIGIKEY: 893-1406-2-ND; MPN: XCL206B183CR-G
U5 = chips:MAX8887: IC REG LDO 3.3V 0.3A TSOT23-5; DIGIKEY: MAX8887EZK33+TCT-ND
U6 = chips:BQ51013B: bq51013B Highly Integrated Wireless Receiver Qi (WPC v1.2) Compliant Power Supply; DIGIKEY: 296-38885-1-ND; MPN: BQ51013B
U7 = chips:NRF52840: ultra-low power 2.4 GHz wireless system on chip (SoC) integrating a multiprotocol 2.4 GHz transceiver, an ARM® Cortex®-M4F CPU.; DIGIKEY: 1490-1071-1-ND; MANUFACTURER: NORIDIC SEMICONDUCTOR; MPN: NRF52840
U8 = chips:SIP32510: Load switch, slew rate controlled. By Vishay; DIGIKEY: SIP32510DT-T1-GE3CT-ND; MANUFACTURER: Vishay; MPN: SIP32510DT-T1-GE3
U9 = switches:SKY13317: Description: Device for SKY13317-373LF, an RF switch from Skyworks Inc.; DATASHEET: http://www.skyworksinc.com/uploads/documents/SKY13317_373LF_200914K.pdf; DESCRIPTION: IC SWITCH RF SP3T 8-MLP; DIGIKEY: 863-1056-1-ND; MANUFACTURER: Skyworks Solutions Inc.; MPN: SKY13317-373LF
U10 = chips:STM32F091CC: Description: STM32F091CC from STMicroelectronics, an ARM-based 32-bit MCU with 256 kB Flash, 32kB of SRAM and a Cortex M0; DATASHEET: https://www.st.com/resource/en/datasheet/stm32f091cc.pdf; DESCRIPTION: IC MCU 32BIT 256KB FLASH 48QFPN; DIGIKEY: 497-15813-ND; MANUFACTURER: STMicroelectronics; MOUSER: 511-STM32F091CCU6; MPN: STM32F091CCU6
U11 = chips:AB1815-T3: Ultra-low current RTC. 55nA quiescent @ 3V. 1.5-3.6V input.; DIGIKEY: 535-11936-1-ND; MANUFACTURER: Abracon; MPN: AB1815-T3
X1 = crystals:ABS05-32.768KHZ: 32.768kHz Crystal; DIGIKEY: 535-11897-1-ND; MANUFACTURER: Abracon; MPN: ABS05-32.768KHZ-9-T
X2 = crystals:FA-20H: Description: Oscillator by EPSON from 12MHz to 54 MHz; DATASHEET: https://support.epson.biz/td/api/doc_check.php?dl=brief_FA-20H_en.pdf; DESCRIPTION: 16MHz ±10ppm Crystal 8pF 80 Ohms 4-SMD, No Lead; DIGIKEY: SER3913CT-ND; MANUFACTURER: EPSON
X3 = crystals:7V: TXC CRYSTAL SMD; DIGIKEY: 887-2568-1-ND; MANUFACTURER: TXC CORPORATION; MPN: 7M-32.000MAHV-T
X4 = crystals:FA-20H: Description: Oscillator by EPSON from 12MHz to 54 MHz; DATASHEET: https://support.epson.biz/td/api/doc_check.php?dl=brief_FA-20H_en.pdf; DESCRIPTION: 38.4MHz ±10ppm Crystal 8.5pF 40 Ohms 4-SMD, No Lead; DIGIKEY: SER3631CT-ND; MANUFACTURER: EPSON
X5 = crystals:ABS07-32.768KHZ: 32.768kHz Crystal; DIGIKEY: 535-9543-1-ND; MANUFACTURER: ABRACON; MPN: ABS07-32.768KHZ-7-T

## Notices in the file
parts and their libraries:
SparkFun-LED: Licensing: CC v3.0 Share-Alike You are welcome to use this library for commercial purposes.
Wurth_Switch_WS-SLSU: Copyright: Würth Elektronik
SparkFun-Jumpers: Licensing: Creative Commons ShareAlike 4.0 International - https://creativecommons.org/licenses/by-sa/4.0
